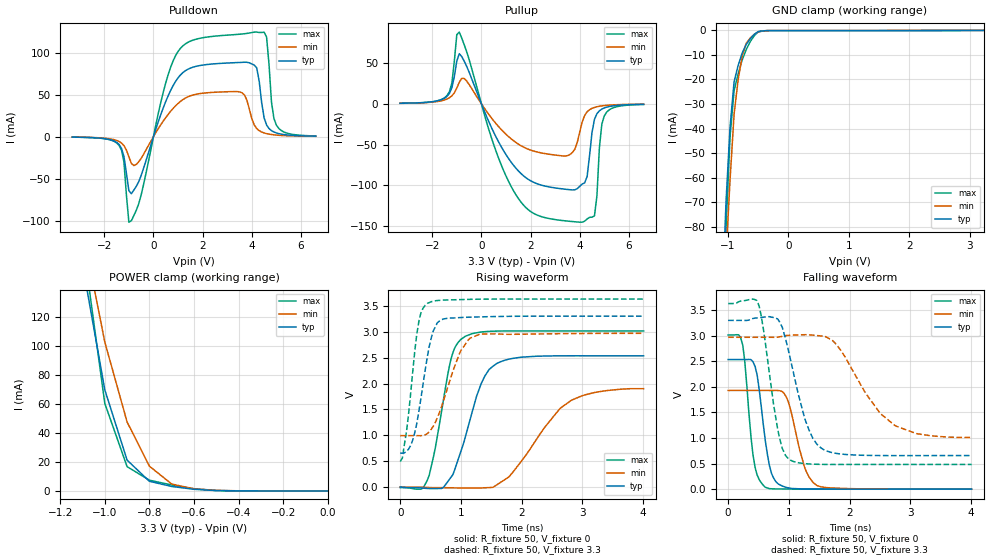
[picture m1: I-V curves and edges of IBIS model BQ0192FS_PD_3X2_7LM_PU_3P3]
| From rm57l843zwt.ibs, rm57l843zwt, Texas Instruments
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|   Model Cell FS_PD_3X2_7LM_PU_3P3
|BQ0192FS_PD_3X2_7LM_PU_3P3
[Model]   BQ0192FS_PD_3X2_7LM_PU_3P3
Model_type   I/O
Polarity   Non-Inverting
Enable   Active-Low
Vinl =  1.25
Vinh =  1.65
Cref =  15.0001pF
Rref =  101.0000M
Vref =  0V
Vmeas =  1.65
C_comp   1.2p   1.2p   1.2p
[Model Spec]
Vinl   1.25   1.12   1.38
Vinh   1.65   1.45   1.75
[Temperature Range]   25   155   -40
[Voltage Range]   3.3   2.97   3.63
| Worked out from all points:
|   slope of the pulldown table from 0 to 0.495 V, typ, clamps not added: 11.9 ohm
|   slope of the pullup table from 0 to 0.495 V, typ, clamps not added: 14.3 ohm
|   GND clamp passes 1 mA (typ) near -0.53 V on its own axis
|   POWER clamp passes 1 mA (typ) near -0.59 V on its own axis
|   rising waveform, R_fixture 50, V_fixture 0: 20-80 % time 400ps typ, 718ps min, 275ps max; typ from 0.001 V to 2.53 V
|   rising waveform, R_fixture 50, V_fixture 3.3: 20-80 % time 224ps typ, 347ps min, 171ps max; typ from 0.657 V to 3.3 V
|   falling waveform, R_fixture 50, V_fixture 0: 20-80 % time 171ps typ, 243ps min, 139ps max; typ from 2.53 V to 0.001 V
|   falling waveform, R_fixture 50, V_fixture 3.3: 20-80 % time 342ps typ, 655ps min, 230ps max; typ from 3.3 V to 0.658 V
[POWER_clamp]
|   voltage   I(typ)   I(min)   I(max)
-3.3V     2.375A     2.63A      3.153A
-1.1V     156mA      180.2mA    173.4mA
-1.067V   127.2mA    154.3mA    135.7mA
-1.033V   98.45mA    128.4mA    97.99mA
-1V       69.65mA    102.5mA    60.28mA
-900mV    21.19mA    47.43mA    16.7mA
-800mV    6.636mA    17.03mA    7.395mA
-700mV    3.052mA    4.718mA    4.065mA
-600mV    1.132mA    1.432mA    1.49mA
-500mV    224.9uA    381.2uA    256.9uA
0V        310pA      5.943nA    270.6pA
[Pulldown]
|   voltage   I(typ)   I(min)   I(max)
-3.3V     -554.3uA   -511.5uA   -526.2uA
-1.4V     -9.291mA   -5.703mA   -10.34mA
-1.2V     -23.68mA   -10.64mA   -30.19mA
-1V       -64.35mA   -24mA      -101.9mA
-600mV    -53.61mA   -29.92mA   -79.97mA
1V        70.16mA    39.6mA     101.5mA
3.5V      88.44mA    53.42mA    122.1mA
4.2V      81.93mA    9.711mA    124.7mA
4.6V      13.96mA    3.646mA    118.8mA
4.8V      7.183mA    2.57mA     41.14mA
5V        4.453mA    1.905mA    13.75mA
6.6V      621.1uA    479.2uA    840.9uA
[Pullup]
|   voltage   I(typ)   I(min)   I(max)
-3.3V     614.6uA    591.9uA    551.1uA
-1.4V     9.028mA    5.738mA    10.01mA
-900mV    61.32mA    26.24mA    87.8mA
1.4V      -78.76mA   -47.33mA   -111.2mA
3.5V      -105mA     -63.56mA   -143.7mA
4.1V      -98.29mA   -22.39mA   -145.1mA
4.3V      -89.13mA   -9.839mA   -141.1mA
4.6V      -19.02mA   -4.469mA   -137.2mA
4.7V      -12.15mA   -3.653mA   -112.5mA
4.8V      -8.616mA   -3.042mA   -53.65mA
5V        -5.089mA   -2.205mA   -14.76mA
6.6V      -663.5uA   -536.5uA   -825.6uA
[GND_clamp]
|   voltage   I(typ)   I(min)   I(max)
-3.3V     -1.947A    -1.623A    -3.254A
-1.1V     -112mA     -127.1mA   -135.8mA
-1.033V   -69.63mA   -91.64mA   -80.2mA
-966.7mV  -39.25mA   -60.63mA   -43.14mA
-900mV    -20.89mA   -34.03mA   -24.56mA
-833.3mV  -14.31mA   -20.14mA   -17.7mA
-766.7mV  -9.259mA   -10.54mA   -12.12mA
-700mV    -5.75mA    -5.239mA   -7.84mA
-566.7mV  -1.652mA   -1.618mA   -2.192mA
-500mV    -488.4uA   -632.2uA   -598.3uA
-300mV    -87.1uA    -54.14uA   -139.1uA
3.233V    -4.592uA   15.73uA    -37.4uA
[Ramp]
| variable   typ   min   max
dV/dt_f   1.631281/0.3491317n   1.216642/0.677392n   1.941456/0.2341526n
dV/dt_r   1.538431/0.4014348n   1.169496/0.7479059n   1.832176/0.2778042n
R_load = 50
[Rising Waveform]
R_fixture = 50
V_fixture = 0
V_fixture_min = 0
V_fixture_max = 0
|   time   V(typ)   V(min)   V(max)
0s        1.041mV    656.3uV    -8.94mV
340ps     -14.27mV   362.3uV    -38.76mV
444ps     -24.74mV   -6.295mV   128.5mV
580ps     -27.81mV   -9.009mV   774.6mV
840ps     199mV      -12.79mV   2.495V
1.072ns   970.5mV    -16.22mV   2.912V
1.332ns   1.996V     -15.29mV   2.995V
1.656ns   2.423V     95.39mV    3.013V
2.808ns   2.535V     1.669V     3.015V
4.008ns   2.534V     1.9V       3.015V
[Rising Waveform]
R_fixture = 50
V_fixture = 3.3
V_fixture_min = 2.97
V_fixture_max = 3.63
|   time   V(typ)   V(min)   V(max)
0s        657.3mV    994.4mV    494.4mV
36ps      656.2mV    994.4mV    564.5mV
104ps     689.1mV    994.4mV    1.083V
204ps     902.9mV    994.5mV    2.207V
308ps     1.473V     993mV      3.208V
444ps     2.5V       1.031V     3.544V
612ps     3.176V     1.341V     3.602V
972ps     3.272V     2.565V     3.619V
1.152ns   3.281V     2.877V     3.625V
4.008ns   3.3V       2.969V     3.63V
[Falling Waveform]
R_fixture = 50
V_fixture = 0
V_fixture_min = 0
V_fixture_max = 0
|   time   V(typ)   V(min)   V(max)
0s        2.534V     1.93V      3.015V
240ps     2.534V     1.93V      2.819V
408ps     2.494V     1.93V      678.1mV
476ps     2.24V      1.93V      281.6mV
612ps     944.5mV    1.93V      36.93mV
716ps     302mV      1.93V      8.51mV
944ps     39.39mV    1.829V     4.204mV
1.256ns   6.41mV     440mV      1.879mV
1.464ns   3.956mV    69.57mV    1.466mV
4.008ns   841uV      1.444mV    803.7uV
[Falling Waveform]
R_fixture = 50
V_fixture = 3.3
V_fixture_min = 2.97
V_fixture_max = 3.63
|   time   V(typ)   V(min)   V(max)
0s        3.3V       2.97V      3.63V
476ps     3.349V     2.97V      3.686V
580ps     3.363V     2.97V      3.133V
816ps     3.327V     2.972V     1.17V
892ps     3.163V     2.99V      795.2mV
1.024ns   2.545V     3.01V      569mV
1.28ns    1.317V     3.021V     498.2mV
1.592ns   758.5mV    2.989V     484.5mV
2.752ns   656.9mV    1.24V      483.6mV
4.008ns   657.6mV    1.011V     483.3mV
